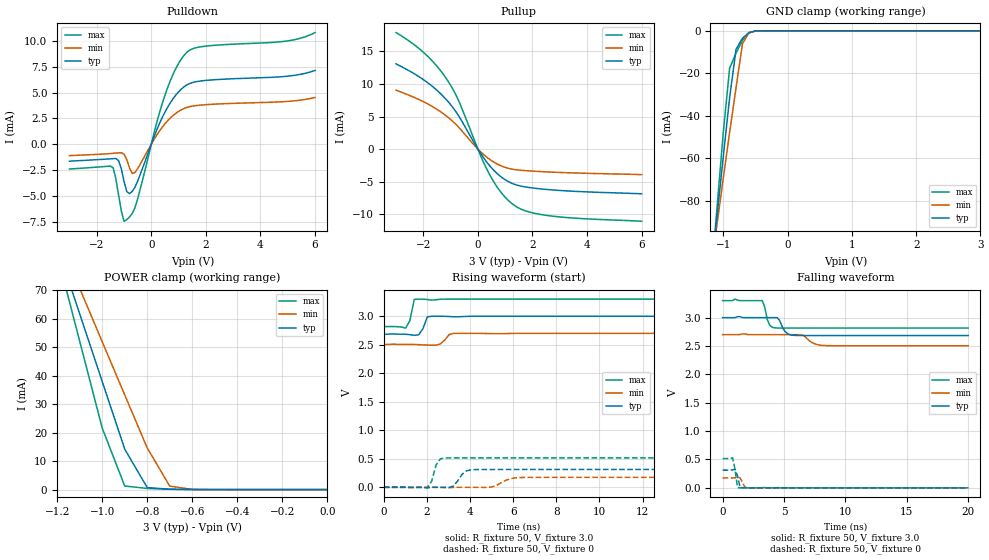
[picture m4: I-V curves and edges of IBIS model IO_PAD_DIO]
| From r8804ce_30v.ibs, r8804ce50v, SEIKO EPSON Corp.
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[Model]   IO_PAD_DIO
Model_type I/O
Enable Active-High
Polarity Non-Inverting
Vinh=2.64
Vinl=0.54
Vmeas=1.50
C_comp   2.5p   2.0p   3.0p
[Temperature Range] 25   105   -40
[Voltage Range]   3.0   2.7   3.3
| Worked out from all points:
|   slope of the pulldown table from 0 to 0.45 V, typ, clamps not added: 158 ohm
|   slope of the pullup table from 0 to 0.45 V, typ, clamps not added: 170 ohm
|   GND clamp passes 1 mA (typ) near -0.61 V on its own axis
|   POWER clamp passes 1 mA (typ) near -0.80 V on its own axis
|   falling waveform, R_fixture 50, V_fixture 3.0: 20-80 % time 463ps typ, 707ps min, 347ps max; typ from 3 V to 2.69 V
|   falling waveform, R_fixture 50, V_fixture 0: 20-80 % time 216ps typ, 254ps min, 226ps max; typ from 0.313 V to 0 V
|   rising waveform, R_fixture 50, V_fixture 3.0: 20-80 % time 216ps typ, 283ps min, 169ps max; typ from 2.69 V to 3 V
|   rising waveform, R_fixture 50, V_fixture 0: 20-80 % time 389ps typ, 559ps min, 249ps max; typ from 0 V to 0.313 V
[Pullup]
-3V       13.09mA    9.053mA    17.89mA
-2V       10.67mA    7.284mA    14.87mA
-1.6V     9.394mA    6.365mA    13.2mA
-1.2V     7.792mA    5.228mA    11.09mA
-700mV    5.066mA    3.34mA     7.375mA
100mV     -669uA     -419.1uA   -1.02mA
400mV     -2.398mA   -1.483mA   -3.684mA
800mV     -4.098mA   -2.481mA   -6.385mA
1.3V      -5.348mA   -3.117mA   -8.539mA
1.8V      -5.848mA   -3.325mA   -9.563mA
2.6V      -6.228mA   -3.518mA   -10.23mA
6V        -6.871mA   -3.923mA   -11.09mA
[Pulldown]
-3V       -1.645mA   -1.105mA   -2.404mA
-1.4V     -1.401mA   -881.9uA   -2.281mA
-1.2V     -1.594mA   -838.2uA   -4.933mA
-1V       -3.61mA    -971.9uA   -7.472mA
-800mV    -4.793mA   -2.307mA   -7.046mA
-600mV    -4.172mA   -2.75mA    -6.158mA
500mV     3.112mA    1.977mA    4.757mA
900mV     4.773mA    3.003mA    7.349mA
1.3V      5.744mA    3.563mA    8.902mA
2V        6.182mA    3.832mA    9.508mA
5V        6.596mA    4.15mA     10.01mA
6V        7.149mA    4.527mA    10.82mA
[GND Clamp]
-3V       -650.3mA   -534.6mA   -803.4mA
-1.2V     -117.3mA   -114.6mA   -121.6mA
-1.1V     -88.33mA   -91.95mA   -84.56mA
-1V       -59.57mA   -69.57mA   -48.26mA
-900mV    -31.49mA   -47.77mA   -17.61mA
-800mV    -8.683mA   -26.7mA    -10.45mA
-700mV    -3.453mA   -6.033mA   -4.512mA
-600mV    -868.8uA   -930.5uA   -956.3uA
-500mV    -86.23uA   -135.6uA   -52.66uA
-400mV    -4.725uA   -14.69uA   -1.074uA
3V        29.22pA    61.44nA    15.58pA
[POWER Clamp]
-3V       518mA      429.9mA    635.9mA
-1.2V     85.6mA     89.47mA    82.67mA
-1.1V     61.75mA    70.7mA     52.12mA
-1V       37.96mA    51.97mA    21.63mA
-900mV    14.22mA    33.28mA    1.266mA
-800mV    725.6uA    14.64mA    407.5uA
-700mV    111.9uA    1.216mA    132.2uA
-600mV    21.56uA    73.28uA    21.07uA
0V        29.22pA    750.2pA    20.24pA
[Falling Waveform]
R_fixture=50
V_fixture=3.0
V_fixture_min=2.7
V_fixture_max=3.3
0s        3V         2.7V       3.3V
3.232ns   3V         2.7V       3.299V
3.838ns   3V         2.7V       2.866V
4.242ns   3.001V     2.7V       2.82V
4.646ns   2.948V     2.7V       2.817V
5.051ns   2.765V     2.7V       2.817V
5.657ns   2.692V     2.7V       2.817V
6.465ns   2.685V     2.699V     2.816V
8.283ns   2.685V     2.509V     2.816V
20ns      2.685V     2.505V     2.816V
[Falling Waveform]
R_fixture=50
V_fixture=0
V_fixture_min=0
V_fixture_max=0
0s        312.9mV    175.1mV    516.2mV
606.1ps   311.1mV    174.2mV    514.5mV
808.1ps   317mV      173.8mV    530.4mV
1.01ns    327.2mV    177.3mV    327.8mV
1.212ns   213.7mV    185.2mV    6.335mV
1.414ns   11.32mV    177.6mV    138.4uV
1.818ns   67.48uV    10.41mV    14.39uV
2.02ns    12.36uV    1.777mV    5.81uV
3.434ns   -3.525uV   332.6nV    5.231mV
20ns      0V         0V         0V
[Rising Waveform]
R_fixture=50
V_fixture=3.0
V_fixture_min=2.7
V_fixture_max=3.3
0s        2.685V     2.505V     2.816V
1.01ns    2.684V     2.506V     2.792V
1.212ns   2.677V     2.505V     2.924V
1.414ns   2.667V     2.505V     3.296V
1.616ns   2.673V     2.502V     3.3V
2.02ns    2.988V     2.494V     3.293V
2.222ns   3V         2.491V     3.283V
2.626ns   3V         2.515V     3.298V
3.232ns   2.99V      2.699V     3.3V
20ns      3V         2.7V       3.3V
[Rising Waveform]
R_fixture=50
V_fixture=0
V_fixture_min=0
V_fixture_max=0
0s        0V         0V         0V
2.02ns    -9.648mV   108.1uV    -1.673mV
2.222ns   -30.29uV   77.84uV    106.2mV
2.424ns   18.82uV    -221.9uV   390.2mV
2.828ns   -1.152mV   -3.426mV   513.3mV
3.232ns   22.03mV    -1.394mV   515.5mV
3.838ns   289.1mV    292.8nV    516.1mV
4.242ns   310.5mV    -358.7uV   516.2mV
6.465ns   312.9mV    172.7mV    516.2mV
20ns      312.9mV    175.1mV    516.2mV
[Ramp]
R_load=50
dV/dt_r   1.877E-1/3.492E-10   1.051E-1/5.346E-10   3.097E-1/2.292E-10
dV/dt_f   1.891E-1/4.429E-10   1.172E-1/7.000E-10   2.901E-1/3.031E-10
|[End   IO_PAD_DIO
